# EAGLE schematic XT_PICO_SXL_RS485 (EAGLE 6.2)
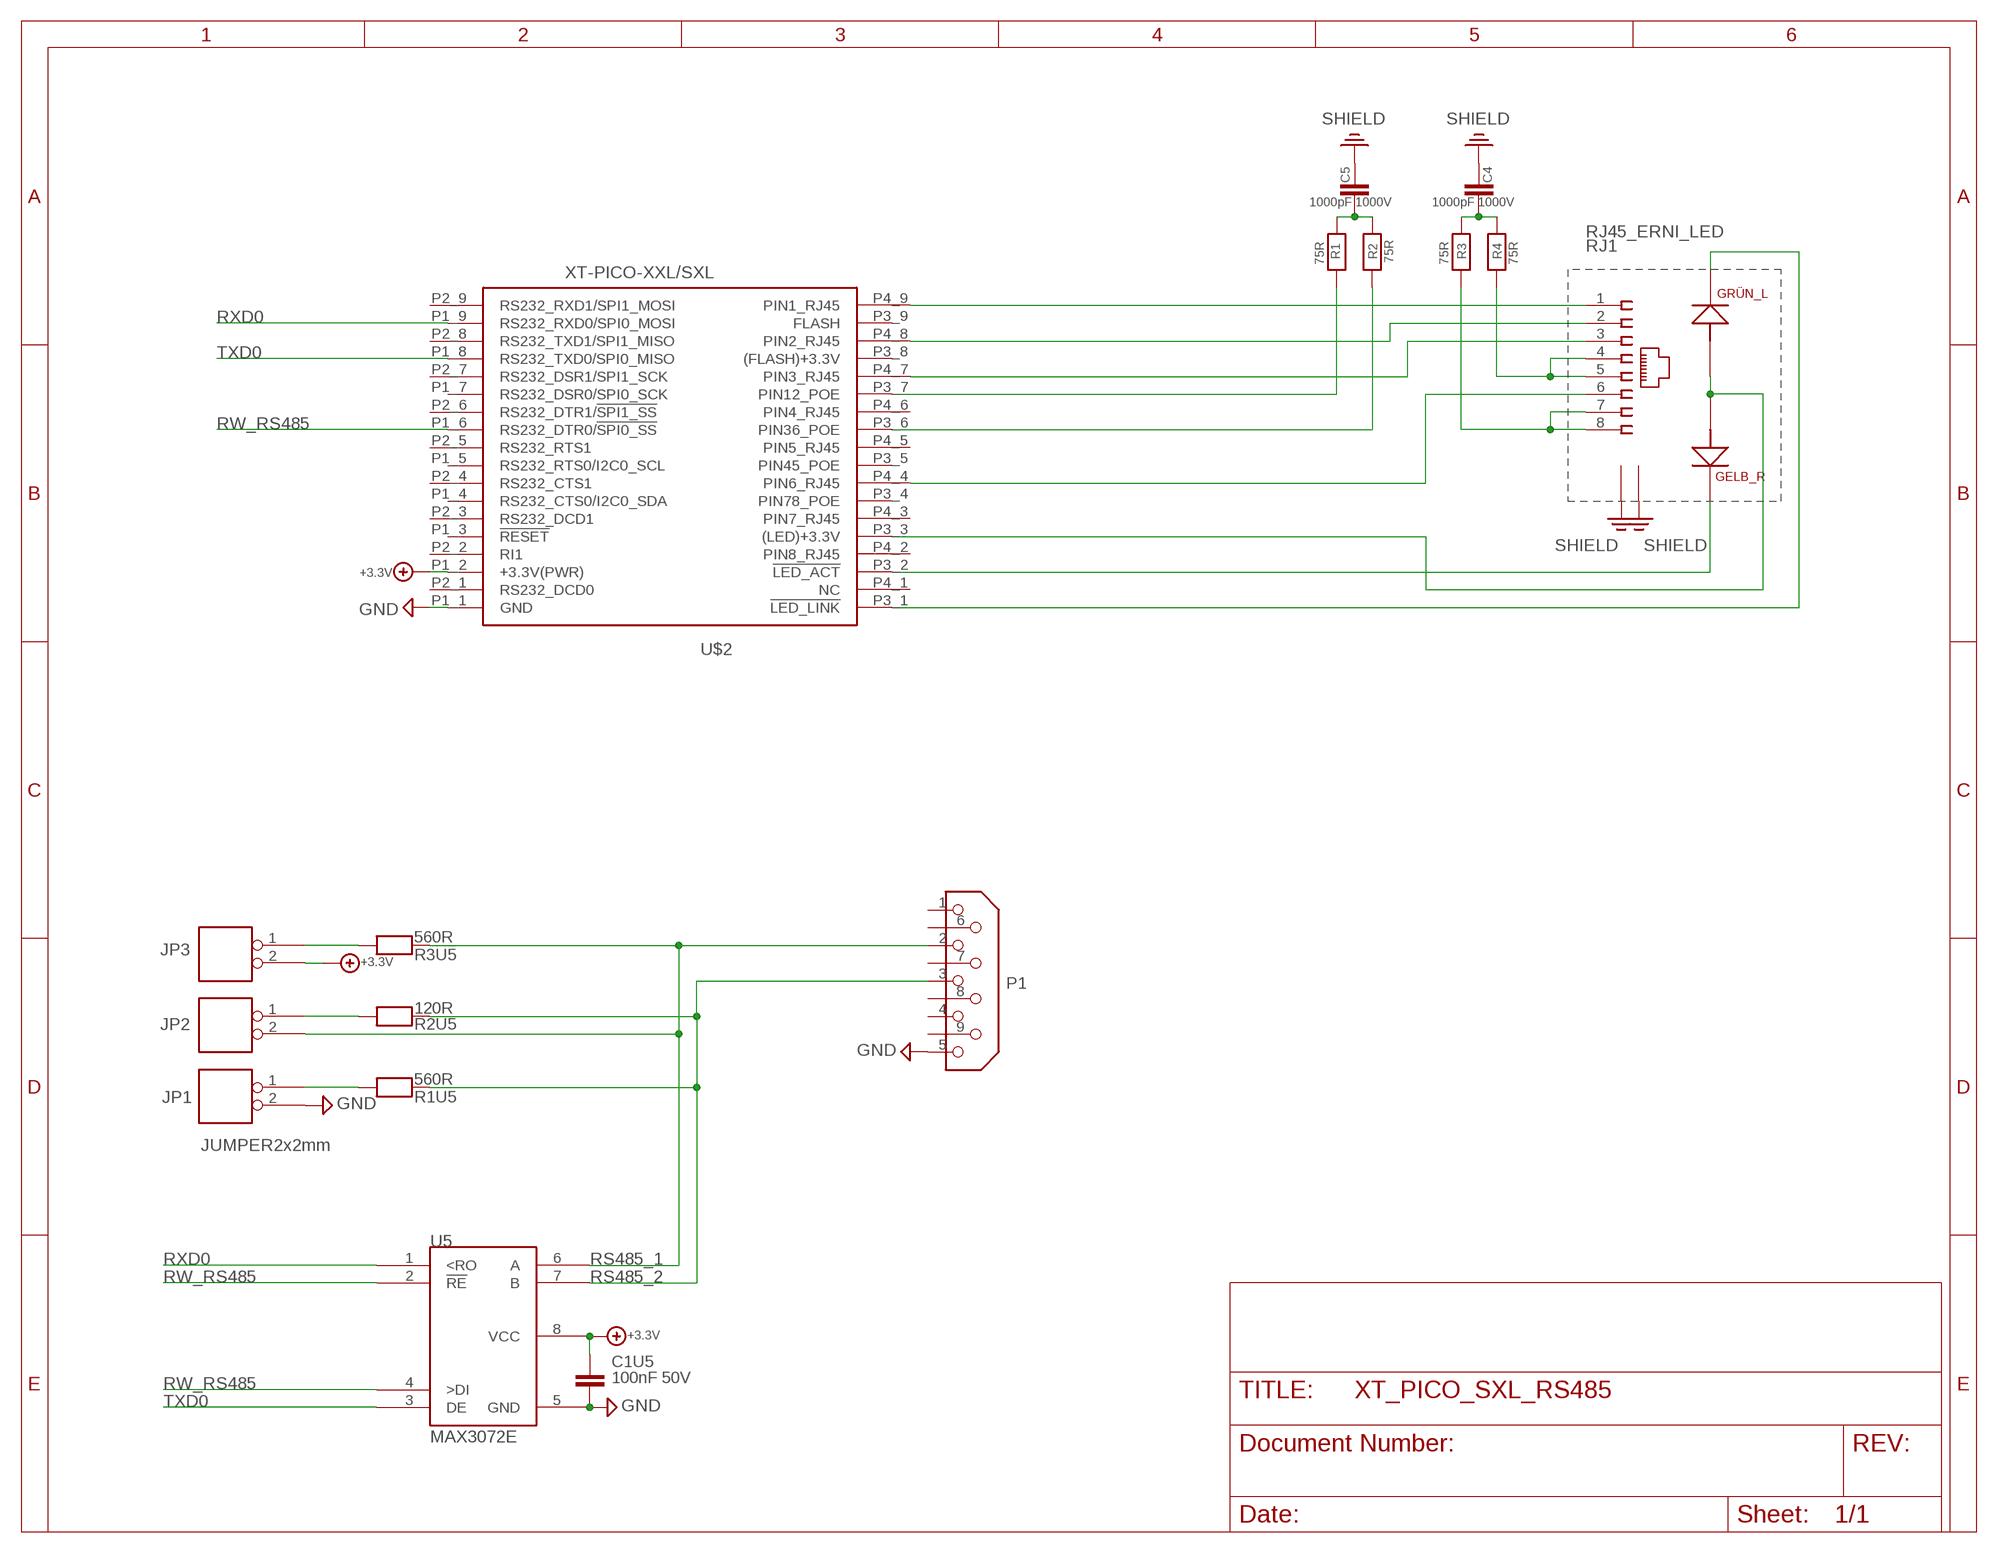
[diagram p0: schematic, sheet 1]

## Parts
C1U5  100nF 50V  CHIP-C-0603  [SMD-0603]
C4  1000pF 1000V  CHIP-C-1210  [SMD-1210]
C5  1000pF 1000V  CHIP-C-1210  [SMD-1210]
JP1  JUMPER2x2mm  JP2  [ROLF_SQW1X2]
JP2  JUMPER2x2mm  JP2  [ROLF_SQW1X2]
JP3  JUMPER2x2mm  JP2  [ROLF_SQW1X2]
P1  DB9  [MSUB9-5]
R1  75R  CHIP-R-0603  [SMD-0603]
R1U5  560R  CHIP-R-0603  [SMD-0603@1]
R2  75R  CHIP-R-0603  [SMD-0603]
R2U5  120R  CHIP-R-0603  [SMD-0603@1]
R3  75R  CHIP-R-0603  [SMD-0603]
R3U5  560R  CHIP-R-0603  [SMD-0603@1]
R4  75R  CHIP-R-0603  [SMD-0603]
RJ1  RJ45_ERNI_LED  [ORCAD_X_ERNI_RJ45_LED]
U5  MAX3072E  MAX3072E_SO8  [SO-8]
U$2  XT-PICO-XXL/SXL  [XT-PICO-XXL/SXL]

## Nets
+3.3V: C1U5.2 JP3.2 U5.8(VCC) U$2.P1_2(+3.3V(PWR))
GND: C1U5.1 JP1.2 P1.5 U5.5(GND) U$2.P1_1(GND)
N14469550: JP2.1 R2U5.2
N15158340: JP1.1 R1U5.2
N15158360: JP3.1 R3U5.2
N$1: R4.2 RJ1.4 RJ1.5
N$2: R3.2 RJ1.7 RJ1.8
N$4: R1.2 U$2.P3_7(PIN12_POE)
N$6: R2.2 U$2.P3_6(PIN36_POE)
N$7: RJ1.1 U$2.P4_9(PIN1_RJ45)
N$8: RJ1.2 U$2.P4_8(PIN2_RJ45)
N$9: RJ1.3 U$2.P4_7(PIN3_RJ45)
N$12: RJ1.6 U$2.P4_4(PIN6_RJ45)
N$15: RJ1.A1 RJ1.A2 U$2.P3_3((LED)+3.3V)
N$16: RJ1.K1 U$2.P3_2(!LED_ACT)
N$17: RJ1.K2 U$2.P3_1(!LED_LINK)
N$19: C4.2 R3.1 R4.1
N$20: C5.1 R1.1 R2.1
PE: RJ1.9 RJ1.10 ; supply symbol labelled SHIELD
RS485_1: JP2.2 P1.2 R3U5.1 U5.6(A)
RS485_2: P1.3 R1U5.1 R2U5.1 U5.7(B)
RW_RS485: U5.2(!RE) U5.4(>DI) U$2.P1_6(RS232_DTR0/!SPI0_SS!)
RXD0: U5.1(<RO) U$2.P1_9(RS232_RXD0/SPI0_MOSI)
SHIELD: C4.1 C5.2
TXD0: U5.3(DE) U$2.P1_8(RS232_TXD0/SPI0_MISO)
Unconnected: P1.1 P1.4 P1.6 P1.7 P1.8 P1.9 U$2.P1_3(!RESET) U$2.P1_4(RS232_CTS0/I2C0_SDA) U$2.P1_5(RS232_RTS0/I2C0_SCL) U$2.P1_7(RS232_DSR0/SPI0_SCK) U$2.P2_1(RS232_DCD0) U$2.P2_2(RI1) U$2.P2_3(RS232_DCD1) U$2.P2_4(RS232_CTS1) U$2.P2_5(RS232_RTS1) U$2.P2_6(RS232_DTR1/!SPI1_SS!) U$2.P2_7(RS232_DSR1/SPI1_SCK) U$2.P2_8(RS232_TXD1/SPI1_MISO) U$2.P2_9(RS232_RXD1/SPI1_MOSI) U$2.P3_4(PIN78_POE) U$2.P3_5(PIN45_POE) U$2.P3_8((FLASH)+3.3V) U$2.P3_9(FLASH) U$2.P4_1(NC) U$2.P4_2(PIN8_RJ45) U$2.P4_3(PIN7_RJ45) U$2.P4_5(PIN5_RJ45) U$2.P4_6(PIN4_RJ45)

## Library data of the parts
C1U5 = mea-lib:CHIP-C-?: Chip capacitance
C4 C5 = XTMACRO:CHIP-C-?: Chip capacitance
JP1-JP3 = XTMACRO_AS:JP2
P1 = XTMACRO:DB9
R1-R4 = XTMACRO:CHIP-R-?: Chip resistors
R1U5 R2U5 R3U5 = mea-lib:CHIP-R-?: Chip resistors
RJ1 = XTMACRO:RJ45_ERNI_LED
U5 = XTMACRO_AS:MAX3072E_SO8
U$2 = ak-devices:XT-PICO-XXL/SXL: AK-NORD XT-PICO-XXL/SXL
